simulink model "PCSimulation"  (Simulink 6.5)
settings: Solver=FixedStepDiscrete  SolverMode=SingleTasking  StartTime=0.0  StopTime=inf  FixedStep=samplePeriod  RelTol=1e-3  AbsTol=1e-6
PreLoadFcn:
  | initialize
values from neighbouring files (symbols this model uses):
  actParams = [	bulkModulus   * pressCanon    [Copy of initialize.m]    (also in initialize.m = [bulkModulus	* pressCanon,)
  displFreq = inf    [initialize.m]
  flowCanon = 1.666667e+04    (= 16666.67)    [Copy of initialize.m]    (also in initialize.m)
  forceCanon = 1    [Copy of initialize.m]    (also in initialize.m)
  forceFreq = inf    [initialize.m]
  friction = 5			 				* 0.155000	 				* 0.00444822 				* area1    (= 2.71252900422)    [initialize.m]
  fsamp = 1 / samplePeriod    (= 1024)    [Copy of initialize.m]    (also in initialize.m; rampth.m = 1 / deltaT; randth.m = 1 / deltaT; rspect.m = 1.0 / tsamp)
  gasConstant = 1.8    [Copy of initialize.m]    (also in initialize.m)
  lengthCanon = 1    [Copy of initialize.m]    (also in initialize.m)
  massCanon = 1e-06    [Copy of initialize.m]    (also in initialize.m)
  maxDispl = ( (stroke2 + endLength2) * lengthCanon)'    [Copy of initialize.m]    (also in initialize.m = 576.2)
  maxOilVolume = volume * (1 - (precharge/supplyPress)^(1/gasConstant))    (= 211.391477114)    [Copy of initialize.m]    (also in initialize.m)
  maxVeloc = ( (maxFlow' * flowCanon ./ (area1 * areaCanon)) / velocCanon)'    [Copy of initialize.m]    (also in initialize.m = (maxFlow * flowCanon / (area1 * areaCanon)) / velocCanon; rampth.m = 2 * maxDispl / (nVeloc * deltaT))
  minDispl = (-(stroke1 + endLength1) * lengthCanon)'    [Copy of initialize.m]    (also in initialize.m = -576.2)
  minVeloc = (-(maxFlow' * flowCanon ./ (area2 * areaCanon)) / velocCanon)'    [Copy of initialize.m]    (also in initialize.m = -(maxFlow * flowCanon / (area2 * areaCanon)) / velocCanon)
  nAct = 5    [Copy of initialize.m]    (also in initialize.m = 1)
  nAdcU = 6    [Copy of initialize.m]    (also in initialize.m = 5)
  nDinp = 4    [Copy of initialize.m]    (also in initialize.m)
  nDout = 4    [Copy of initialize.m]    (also in initialize.m)
  nDucU = 2    [Copy of initialize.m]    (also in initialize.m)
  nEncU = 3    [Copy of initialize.m]    (also in initialize.m)
  nUDPInp = 1+6*nAct+nAdcU+nDucU+nEncU+nDout    (= 46)    [Copy of initialize.m]    (also in initialize.m = 10)
  nUDPOut = 1+7*nAct+nAdcU+nDucU+nEncU+nDinp    (= 51)    [Copy of initialize.m]    (also in initialize.m = 12)
  precharge = 3000		 				* 6.894757e-03    (= 20.684271)    [Copy of initialize.m]    (also in initialize.m)
  pumpFlow = 1e20    (= 1e+20)    [Copy of initialize.m]    (also in initialize.m)
  returnPress = 3			 				* 0.1    (= 0.3)    [Copy of initialize.m]    (also in initialize.m)
  samplePeriod = controlPeriod/upsampleFactor    (= 0.0009765625)    [Copy of initialize.m]    (also in initialize.m; viewer.m = eval(getHeaderValue(header, 'DELTA_T')))
  springCanon = 1    [Copy of initialize.m]    (also in initialize.m)
  supplyPress = 280		 				* 0.1    (= 28)    [Copy of initialize.m]    (also in initialize.m)
  upsampleFactor = 1    [Copy of initialize.m]    (also in initialize.m)
  velocCanon = 1    [Copy of initialize.m]    (also in initialize.m)
  volume = 15.15		 				+ (  45		 				    * 2		 				   + 30		 				    * 6 )	 				* 5    (= 1365.15)    [Copy of initialize.m]    (also in initialize.m; quake.m = volume / 231.0)
  volumeCanon = 1e+06    (= 1000000)    [Copy of initialize.m]    (also in initialize.m)
  yieldDispl = 1.0    (= 1)    [initialize.m]
undefined symbols (not defined in the file or in its folder): DiscIntNeverNeededParam, dpforceFreq, mass, spring, staticForce
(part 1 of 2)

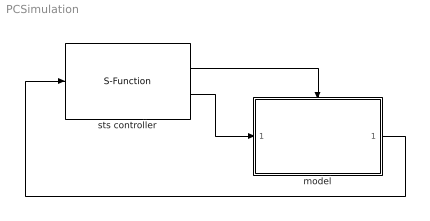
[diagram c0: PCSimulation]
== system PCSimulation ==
  model : Subsystem  TreatAsAtomicUnit=on
  sts controller : S-Function  FunctionName=ConnectUdpSimulink  Parameters=5002,nUDPInp,nUDPOut,upsampleFactor
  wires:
  model/1(out) -> sts controller/1
  sts controller/1 -> model/Trigger
  sts controller/2 -> model/1(inp)

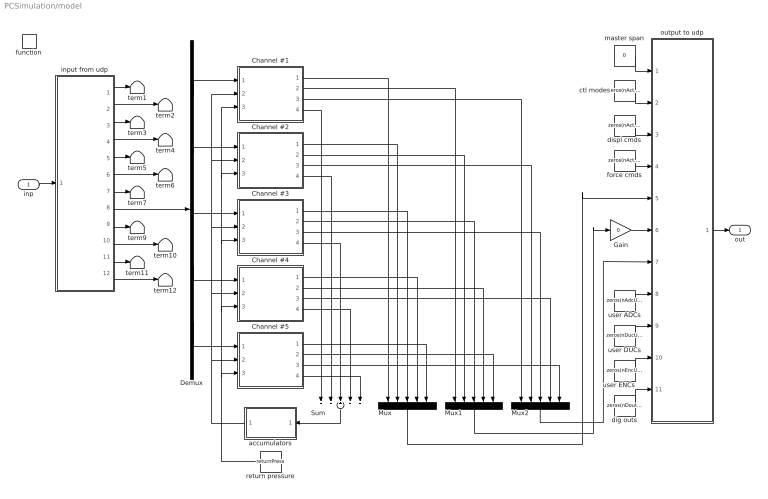
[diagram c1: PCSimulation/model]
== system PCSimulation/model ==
  inp : Inport
  function : TriggerPort  TriggerType=function-call
  Channel #1 : Subsystem  mask{id=1}
      mask prompts: id "Channel ID"
  Channel #2 : Subsystem  mask{id=2}
      mask prompts: id "Channel ID"
  Channel #3 : Subsystem  mask{id=3}
      mask prompts: id "Channel ID"
  Channel #4 : Subsystem  mask{id=4}
      mask prompts: id "Channel ID"
  Channel #5 : Subsystem  mask{id=5}
      mask prompts: id "Channel ID"
  Demux : Demux  Outputs=nAct
  Gain : Gain  Gain=0
  Mux : Mux  Orientation=down  Inputs=nAct
  Mux1 : Mux  Orientation=down  Inputs=nAct
  Mux2 : Mux  Orientation=down  Inputs=nAct
  Sum : Sum  Orientation=down  Inputs=+++++
  accumulators : Subsystem  Orientation=left
  ctl modes : Constant  Value=zeros(nAct, 1)  OutDataType=sfix(16)  ConRadixGroup=Use specified scaling  OutScaling=2^0  SampleTime=inf  FramePeriod=inf
  dig outs : Constant  Value=zeros(nDout, 1)  OutDataTypeMode=uint32  OutDataType=sfix(16)  ConRadixGroup=Use specified scaling  OutScaling=2^0  SampleTime=inf  FramePeriod=inf
  displ cmds : Constant  Value=zeros(nAct, 1)  OutDataType=sfix(16)  ConRadixGroup=Use specified scaling  OutScaling=2^0  SampleTime=inf  FramePeriod=inf
  force cmds : Constant  Value=zeros(nAct, 1)  OutDataType=sfix(16)  ConRadixGroup=Use specified scaling  OutScaling=2^0  SampleTime=inf  FramePeriod=inf
  input from udp : Subsystem
  master span : Constant  Value=0  OutDataType=sfix(16)  ConRadixGroup=Use specified scaling  OutScaling=2^0  SampleTime=inf  FramePeriod=inf
  output to udp : Subsystem
  return pressure : Constant  Orientation=left  Value=returnPress  OutDataType=sfix(16)  ConRadixGroup=Use specified scaling  OutScaling=2^0  SampleTime=inf  FramePeriod=inf
  term{1..7,9..12} (11 alike) : Terminator
  user ADCs : Constant  Value=zeros(nAdcU, 1)  OutDataType=sfix(16)  ConRadixGroup=Use specified scaling  OutScaling=2^0  SampleTime=inf  FramePeriod=inf
  user DUCs : Constant  Value=zeros(nDucU, 1)  OutDataType=sfix(16)  ConRadixGroup=Use specified scaling  OutScaling=2^0  SampleTime=inf  FramePeriod=inf
  user ENCs : Constant  Value=zeros(nEncU, 1)  OutDataType=sfix(16)  ConRadixGroup=Use specified scaling  OutScaling=2^0  SampleTime=inf  FramePeriod=inf
  out : Outport
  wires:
  input from udp/3(displ cmds) -> term3/1
  input from udp/1(master span) -> term1/1
  input from udp/6(force fbks) -> term6/1
  input from udp/10(user ducs) -> term10/1
  input from udp/12(dig inps) -> term12/1
  input from udp/2(ctl modes) -> term2/1
  input from udp/4(force cmds) -> term4/1
  input from udp/5(displ fbks) -> term5/1
  input from udp/7(dpforce fbks) -> term7/1
  input from udp/9(user adcs) -> term9/1
  input from udp/11(user encs) -> term11/1
  inp/1 -> input from udp/1(inp)
  master span/1 -> output to udp/1(master span)
  ctl modes/1 -> output to udp/2(ctl modes)
  displ cmds/1 -> output to udp/3(displ cmds)
  force cmds/1 -> output to udp/4(force cmds)
  user ADCs/1 -> output to udp/8(user adcs)
  user DUCs/1 -> output to udp/9(user ducs)
  user ENCs/1 -> output to udp/10(user encs)
  dig outs/1 -> output to udp/11(dig outs)
  output to udp/1(out) -> out/1
  Channel #1/4(flow) -> Sum/1
  Channel #2/4(flow) -> Sum/2
  Channel #3/4(flow) -> Sum/3
  Sum/1 -> accumulators/1(flow)
  Channel #4/4(flow) -> Sum/4
  Channel #5/4(flow) -> Sum/5
  Channel #1/1(displ) -> Mux/1
  Channel #2/1(displ) -> Mux/2
  Channel #3/1(displ) -> Mux/3
  Channel #4/1(displ) -> Mux/4
  Channel #5/1(displ) -> Mux/5
  Channel #1/2(force) -> Mux1/1
  Channel #2/2(force) -> Mux1/2
  Channel #3/2(force) -> Mux1/3
  Channel #4/2(force) -> Mux1/4
  Channel #5/2(force) -> Mux1/5
  Channel #1/3(dpforce) -> Mux2/1
  Channel #2/3(dpforce) -> Mux2/2
  Channel #3/3(dpforce) -> Mux2/3
  Channel #4/3(dpforce) -> Mux2/4
  Channel #5/3(dpforce) -> Mux2/5
  Mux/1 -> output to udp/5(displ fbks)
  Mux1/1 -> Gain/1
  Mux2/1 -> output to udp/7(dpforce fbks)
  input from udp/8(valve cmds) -> Demux/1
  Demux/1 -> Channel #1/1(valve cmd)
  Demux/2 -> Channel #2/1(valve cmd)
  Demux/3 -> Channel #3/1(valve cmd)
  Demux/4 -> Channel #4/1(valve cmd)
  Demux/5 -> Channel #5/1(valve cmd)
  accumulators/1(press) -> Channel #1/2(spl press), Channel #2/2(spl press), Channel #3/2(spl press), Channel #4/2(spl press), Channel #5/2(spl press)
  return pressure/1 -> Channel #1/3(rtn press), Channel #2/3(rtn press), Channel #3/3(rtn press), Channel #4/3(rtn press), Channel #5/3(rtn press)
  Gain/1 -> output to udp/6(force fbks)

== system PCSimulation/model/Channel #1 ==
  valve cmd : Inport
  spl press : Inport  Port=2
  rtn press : Inport  Port=3
  displ cond filter : Subsystem  mask{freq3dB=displFreq(id), fsamp=fsamp}
      mask prompts: freq3dB "3 dB cutoff frequency (inf, 500, 300, 100, 50 Hz)"; fsamp "Sampling frequency (Hz)"
      mask init:
      | if isempty(freq3dB)
      | 	freq3dB = fsamp;
      | elseif freq3dB == 500
      | 	freq3dB = 485;
      | elseif freq3dB == 300
      | 	freq3dB = 204.9;
      | elseif freq3dB == 100
      | 	freq3dB = 56.5;
      | elseif freq3dB == 50
      | 	freq3dB = 27.8;
      | else
      | 	freq3dB = fsamp;
      | end
      | if freq3dB > fsamp/2
      | 	a = [1];
      | 	b = [1];
      | else
      | 	[b, a] = ellip(4, 0.001, 60.0, 2*freq3dB/fsamp);
      | end
  dpforce cond filter : Subsystem  mask{freq3dB=dpforceFreq(id), fsamp=fsamp}
      mask prompts: freq3dB "3 dB cutoff frequency (inf, 500, 300, 100, 50 Hz)"; fsamp "Sampling frequency (Hz)"
      mask init:
      | if isempty(freq3dB)
      | 	freq3dB = fsamp;
      | elseif freq3dB == 500
      | 	freq3dB = 485;
      | elseif freq3dB == 300
      | 	freq3dB = 204.9;
      | elseif freq3dB == 100
      | 	freq3dB = 56.5;
      | elseif freq3dB == 50
      | 	freq3dB = 27.8;
      | else
      | 	freq3dB = fsamp;
      | end
      | if freq3dB > fsamp/2
      | 	a = [1];
      | 	b = [1];
      | else
      | 	[b, a] = ellip(4, 0.001, 60.0, 2*freq3dB/fsamp);
      | end
  force cond filter : Subsystem  mask{freq3dB=forceFreq((id)), fsamp=fsamp}
      mask prompts: freq3dB "3 dB cutoff frequency (inf, 500, 300, 100, 50 Hz)"; fsamp "Sampling frequency (Hz)"
      mask init:
      | if isempty(freq3dB)
      | 	freq3dB = fsamp;
      | elseif freq3dB == 500
      | 	freq3dB = 485;
      | elseif freq3dB == 300
      | 	freq3dB = 204.9;
      | elseif freq3dB == 100
      | 	freq3dB = 56.5;
      | elseif freq3dB == 50
      | 	freq3dB = 27.8;
      | else
      | 	freq3dB = fsamp;
      | end
      | if freq3dB > fsamp/2
      | 	a = [1];
      | 	b = [1];
      | else
      | 	[b, a] = ellip(4, 0.001, 60.0, 2*freq3dB/fsamp);
      | end
  payload : Subsystem
  servovalve & actuator : Subsystem  mask(Actuator){params=actParams(:,id)}
      mask prompts: params "Parameter vector"
  displ : Outport
  force : Outport  Port=2
  dpforce : Outport  Port=3
  flow : Outport  Port=4
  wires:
  payload/2(veloc) -> servovalve & actuator/3(veloc)
  payload/1(displ) -> displ cond filter/1(inp), servovalve & actuator/2(displ)
  valve cmd/1 -> servovalve & actuator/1(cmd)
  rtn press/1 -> servovalve & actuator/5(rtn press)
  spl press/1 -> servovalve & actuator/4(spl press)
  servovalve & actuator/2(flow) -> flow/1
  servovalve & actuator/1(force) -> force cond filter/1(inp), dpforce cond filter/1(inp), payload/1(force)
  displ cond filter/1(out) -> displ/1
  force cond filter/1(out) -> force/1
  dpforce cond filter/1(out) -> dpforce/1

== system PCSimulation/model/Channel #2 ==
  valve cmd : Inport
  spl press : Inport  Port=2
  rtn press : Inport  Port=3
  displ cond filter : Subsystem  mask{freq3dB=displFreq(id), fsamp=fsamp}
      mask prompts: freq3dB "3 dB cutoff frequency (inf, 500, 300, 100, 50 Hz)"; fsamp "Sampling frequency (Hz)"
      mask init:
      | if isempty(freq3dB)
      | 	freq3dB = fsamp;
      | elseif freq3dB == 500
      | 	freq3dB = 485;
      | elseif freq3dB == 300
      | 	freq3dB = 204.9;
      | elseif freq3dB == 100
      | 	freq3dB = 56.5;
      | elseif freq3dB == 50
      | 	freq3dB = 27.8;
      | else
      | 	freq3dB = fsamp;
      | end
      | if freq3dB > fsamp/2
      | 	a = [1];
      | 	b = [1];
      | else
      | 	[b, a] = ellip(4, 0.001, 60.0, 2*freq3dB/fsamp);
      | end
  dpforce cond filter : Subsystem  mask{freq3dB=dpforceFreq(id), fsamp=fsamp}
      mask prompts: freq3dB "3 dB cutoff frequency (inf, 500, 300, 100, 50 Hz)"; fsamp "Sampling frequency (Hz)"
      mask init:
      | if isempty(freq3dB)
      | 	freq3dB = fsamp;
      | elseif freq3dB == 500
      | 	freq3dB = 485;
      | elseif freq3dB == 300
      | 	freq3dB = 204.9;
      | elseif freq3dB == 100
      | 	freq3dB = 56.5;
      | elseif freq3dB == 50
      | 	freq3dB = 27.8;
      | else
      | 	freq3dB = fsamp;
      | end
      | if freq3dB > fsamp/2
      | 	a = [1];
      | 	b = [1];
      | else
      | 	[b, a] = ellip(4, 0.001, 60.0, 2*freq3dB/fsamp);
      | end
  force cond filter : Subsystem  mask{freq3dB=forceFreq((id)), fsamp=fsamp}
      mask prompts: freq3dB "3 dB cutoff frequency (inf, 500, 300, 100, 50 Hz)"; fsamp "Sampling frequency (Hz)"
      mask init:
      | if isempty(freq3dB)
      | 	freq3dB = fsamp;
      | elseif freq3dB == 500
      | 	freq3dB = 485;
      | elseif freq3dB == 300
      | 	freq3dB = 204.9;
      | elseif freq3dB == 100
      | 	freq3dB = 56.5;
      | elseif freq3dB == 50
      | 	freq3dB = 27.8;
      | else
      | 	freq3dB = fsamp;
      | end
      | if freq3dB > fsamp/2
      | 	a = [1];
      | 	b = [1];
      | else
      | 	[b, a] = ellip(4, 0.001, 60.0, 2*freq3dB/fsamp);
      | end
  payload : Subsystem
  servovalve & actuator : Subsystem  mask(Actuator){params=actParams(:,id)}
      mask prompts: params "Parameter vector"
  displ : Outport
  force : Outport  Port=2
  dpforce : Outport  Port=3
  flow : Outport  Port=4
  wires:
  dpforce cond filter/1(out) -> dpforce/1
  force cond filter/1(out) -> force/1
  displ cond filter/1(out) -> displ/1
  servovalve & actuator/1(force) -> payload/1(force), dpforce cond filter/1(inp), force cond filter/1(inp)
  servovalve & actuator/2(flow) -> flow/1
  spl press/1 -> servovalve & actuator/4(spl press)
  rtn press/1 -> servovalve & actuator/5(rtn press)
  valve cmd/1 -> servovalve & actuator/1(cmd)
  payload/1(displ) -> servovalve & actuator/2(displ), displ cond filter/1(inp)
  payload/2(veloc) -> servovalve & actuator/3(veloc)

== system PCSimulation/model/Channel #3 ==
  valve cmd : Inport
  spl press : Inport  Port=2
  rtn press : Inport  Port=3
  displ cond filter : Subsystem  mask{freq3dB=displFreq(id), fsamp=fsamp}
      mask prompts: freq3dB "3 dB cutoff frequency (inf, 500, 300, 100, 50 Hz)"; fsamp "Sampling frequency (Hz)"
      mask init:
      | if isempty(freq3dB)
      | 	freq3dB = fsamp;
      | elseif freq3dB == 500
      | 	freq3dB = 485;
      | elseif freq3dB == 300
      | 	freq3dB = 204.9;
      | elseif freq3dB == 100
      | 	freq3dB = 56.5;
      | elseif freq3dB == 50
      | 	freq3dB = 27.8;
      | else
      | 	freq3dB = fsamp;
      | end
      | if freq3dB > fsamp/2
      | 	a = [1];
      | 	b = [1];
      | else
      | 	[b, a] = ellip(4, 0.001, 60.0, 2*freq3dB/fsamp);
      | end
  dpforce cond filter : Subsystem  mask{freq3dB=dpforceFreq(id), fsamp=fsamp}
      mask prompts: freq3dB "3 dB cutoff frequency (inf, 500, 300, 100, 50 Hz)"; fsamp "Sampling frequency (Hz)"
      mask init:
      | if isempty(freq3dB)
      | 	freq3dB = fsamp;
      | elseif freq3dB == 500
      | 	freq3dB = 485;
      | elseif freq3dB == 300
      | 	freq3dB = 204.9;
      | elseif freq3dB == 100
      | 	freq3dB = 56.5;
      | elseif freq3dB == 50
      | 	freq3dB = 27.8;
      | else
      | 	freq3dB = fsamp;
      | end
      | if freq3dB > fsamp/2
      | 	a = [1];
      | 	b = [1];
      | else
      | 	[b, a] = ellip(4, 0.001, 60.0, 2*freq3dB/fsamp);
      | end
  force cond filter : Subsystem  mask{freq3dB=forceFreq((id)), fsamp=fsamp}
      mask prompts: freq3dB "3 dB cutoff frequency (inf, 500, 300, 100, 50 Hz)"; fsamp "Sampling frequency (Hz)"
      mask init:
      | if isempty(freq3dB)
      | 	freq3dB = fsamp;
      | elseif freq3dB == 500
      | 	freq3dB = 485;
      | elseif freq3dB == 300
      | 	freq3dB = 204.9;
      | elseif freq3dB == 100
      | 	freq3dB = 56.5;
      | elseif freq3dB == 50
      | 	freq3dB = 27.8;
      | else
      | 	freq3dB = fsamp;
      | end
      | if freq3dB > fsamp/2
      | 	a = [1];
      | 	b = [1];
      | else
      | 	[b, a] = ellip(4, 0.001, 60.0, 2*freq3dB/fsamp);
      | end
  payload : Subsystem
  servovalve & actuator : Subsystem  mask(Actuator){params=actParams(:,id)}
      mask prompts: params "Parameter vector"
  displ : Outport
  force : Outport  Port=2
  dpforce : Outport  Port=3
  flow : Outport  Port=4
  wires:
  payload/2(veloc) -> servovalve & actuator/3(veloc)
  payload/1(displ) -> displ cond filter/1(inp), servovalve & actuator/2(displ)
  valve cmd/1 -> servovalve & actuator/1(cmd)
  rtn press/1 -> servovalve & actuator/5(rtn press)
  spl press/1 -> servovalve & actuator/4(spl press)
  servovalve & actuator/2(flow) -> flow/1
  servovalve & actuator/1(force) -> force cond filter/1(inp), dpforce cond filter/1(inp), payload/1(force)
  displ cond filter/1(out) -> displ/1
  force cond filter/1(out) -> force/1
  dpforce cond filter/1(out) -> dpforce/1

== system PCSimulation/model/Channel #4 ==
  valve cmd : Inport
  spl press : Inport  Port=2
  rtn press : Inport  Port=3
  displ cond filter : Subsystem  mask{freq3dB=displFreq(id), fsamp=fsamp}
      mask prompts: freq3dB "3 dB cutoff frequency (inf, 500, 300, 100, 50 Hz)"; fsamp "Sampling frequency (Hz)"
      mask init:
      | if isempty(freq3dB)
      | 	freq3dB = fsamp;
      | elseif freq3dB == 500
      | 	freq3dB = 485;
      | elseif freq3dB == 300
      | 	freq3dB = 204.9;
      | elseif freq3dB == 100
      | 	freq3dB = 56.5;
      | elseif freq3dB == 50
      | 	freq3dB = 27.8;
      | else
      | 	freq3dB = fsamp;
      | end
      | if freq3dB > fsamp/2
      | 	a = [1];
      | 	b = [1];
      | else
      | 	[b, a] = ellip(4, 0.001, 60.0, 2*freq3dB/fsamp);
      | end
  dpforce cond filter : Subsystem  mask{freq3dB=dpforceFreq(id), fsamp=fsamp}
      mask prompts: freq3dB "3 dB cutoff frequency (inf, 500, 300, 100, 50 Hz)"; fsamp "Sampling frequency (Hz)"
      mask init:
      | if isempty(freq3dB)
      | 	freq3dB = fsamp;
      | elseif freq3dB == 500
      | 	freq3dB = 485;
      | elseif freq3dB == 300
      | 	freq3dB = 204.9;
      | elseif freq3dB == 100
      | 	freq3dB = 56.5;
      | elseif freq3dB == 50
      | 	freq3dB = 27.8;
      | else
      | 	freq3dB = fsamp;
      | end
      | if freq3dB > fsamp/2
      | 	a = [1];
      | 	b = [1];
      | else
      | 	[b, a] = ellip(4, 0.001, 60.0, 2*freq3dB/fsamp);
      | end
  force cond filter : Subsystem  mask{freq3dB=forceFreq((id)), fsamp=fsamp}
      mask prompts: freq3dB "3 dB cutoff frequency (inf, 500, 300, 100, 50 Hz)"; fsamp "Sampling frequency (Hz)"
      mask init:
      | if isempty(freq3dB)
      | 	freq3dB = fsamp;
      | elseif freq3dB == 500
      | 	freq3dB = 485;
      | elseif freq3dB == 300
      | 	freq3dB = 204.9;
      | elseif freq3dB == 100
      | 	freq3dB = 56.5;
      | elseif freq3dB == 50
      | 	freq3dB = 27.8;
      | else
      | 	freq3dB = fsamp;
      | end
      | if freq3dB > fsamp/2
      | 	a = [1];
      | 	b = [1];
      | else
      | 	[b, a] = ellip(4, 0.001, 60.0, 2*freq3dB/fsamp);
      | end
  payload : Subsystem
  servovalve & actuator : Subsystem  mask(Actuator){params=actParams(:,id)}
      mask prompts: params "Parameter vector"
  displ : Outport
  force : Outport  Port=2
  dpforce : Outport  Port=3
  flow : Outport  Port=4
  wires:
  dpforce cond filter/1(out) -> dpforce/1
  force cond filter/1(out) -> force/1
  displ cond filter/1(out) -> displ/1
  servovalve & actuator/1(force) -> payload/1(force), dpforce cond filter/1(inp), force cond filter/1(inp)
  servovalve & actuator/2(flow) -> flow/1
  spl press/1 -> servovalve & actuator/4(spl press)
  rtn press/1 -> servovalve & actuator/5(rtn press)
  valve cmd/1 -> servovalve & actuator/1(cmd)
  payload/1(displ) -> servovalve & actuator/2(displ), displ cond filter/1(inp)
  payload/2(veloc) -> servovalve & actuator/3(veloc)

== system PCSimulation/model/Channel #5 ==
  valve cmd : Inport
  spl press : Inport  Port=2
  rtn press : Inport  Port=3
  displ cond filter : Subsystem  mask{freq3dB=displFreq(id), fsamp=fsamp}
      mask prompts: freq3dB "3 dB cutoff frequency (inf, 500, 300, 100, 50 Hz)"; fsamp "Sampling frequency (Hz)"
      mask init:
      | if isempty(freq3dB)
      | 	freq3dB = fsamp;
      | elseif freq3dB == 500
      | 	freq3dB = 485;
      | elseif freq3dB == 300
      | 	freq3dB = 204.9;
      | elseif freq3dB == 100
      | 	freq3dB = 56.5;
      | elseif freq3dB == 50
      | 	freq3dB = 27.8;
      | else
      | 	freq3dB = fsamp;
      | end
      | if freq3dB > fsamp/2
      | 	a = [1];
      | 	b = [1];
      | else
      | 	[b, a] = ellip(4, 0.001, 60.0, 2*freq3dB/fsamp);
      | end
  dpforce cond filter : Subsystem  mask{freq3dB=dpforceFreq(id), fsamp=fsamp}
      mask prompts: freq3dB "3 dB cutoff frequency (inf, 500, 300, 100, 50 Hz)"; fsamp "Sampling frequency (Hz)"
      mask init:
      | if isempty(freq3dB)
      | 	freq3dB = fsamp;
      | elseif freq3dB == 500
      | 	freq3dB = 485;
      | elseif freq3dB == 300
      | 	freq3dB = 204.9;
      | elseif freq3dB == 100
      | 	freq3dB = 56.5;
      | elseif freq3dB == 50
      | 	freq3dB = 27.8;
      | else
      | 	freq3dB = fsamp;
      | end
      | if freq3dB > fsamp/2
      | 	a = [1];
      | 	b = [1];
      | else
      | 	[b, a] = ellip(4, 0.001, 60.0, 2*freq3dB/fsamp);
      | end
  force cond filter : Subsystem  mask{freq3dB=forceFreq((id)), fsamp=fsamp}
      mask prompts: freq3dB "3 dB cutoff frequency (inf, 500, 300, 100, 50 Hz)"; fsamp "Sampling frequency (Hz)"
      mask init:
      | if isempty(freq3dB)
      | 	freq3dB = fsamp;
      | elseif freq3dB == 500
      | 	freq3dB = 485;
      | elseif freq3dB == 300
      | 	freq3dB = 204.9;
      | elseif freq3dB == 100
      | 	freq3dB = 56.5;
      | elseif freq3dB == 50
      | 	freq3dB = 27.8;
      | else
      | 	freq3dB = fsamp;
      | end
      | if freq3dB > fsamp/2
      | 	a = [1];
      | 	b = [1];
      | else
      | 	[b, a] = ellip(4, 0.001, 60.0, 2*freq3dB/fsamp);
      | end
  payload : Subsystem
  servovalve & actuator : Subsystem  mask(Actuator){params=actParams(:,id)}
      mask prompts: params "Parameter vector"
  displ : Outport
  force : Outport  Port=2
  dpforce : Outport  Port=3
  flow : Outport  Port=4
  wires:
  payload/2(veloc) -> servovalve & actuator/3(veloc)
  payload/1(displ) -> displ cond filter/1(inp), servovalve & actuator/2(displ)
  valve cmd/1 -> servovalve & actuator/1(cmd)
  rtn press/1 -> servovalve & actuator/5(rtn press)
  spl press/1 -> servovalve & actuator/4(spl press)
  servovalve & actuator/2(flow) -> flow/1
  servovalve & actuator/1(force) -> force cond filter/1(inp), dpforce cond filter/1(inp), payload/1(force)
  displ cond filter/1(out) -> displ/1
  force cond filter/1(out) -> force/1
  dpforce cond filter/1(out) -> dpforce/1

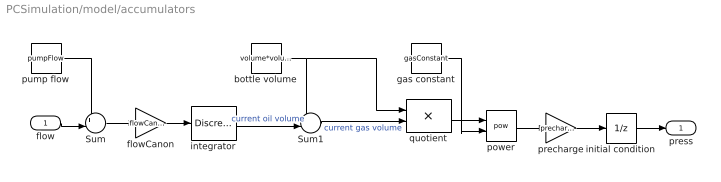
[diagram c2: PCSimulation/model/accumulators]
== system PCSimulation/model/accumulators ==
  flow : Inport
  Sum : Sum  Inputs=+-|
  Sum1 : Sum  Inputs=+-|
  bottle volume : Constant  Value=volume*volumeCanon  OutDataType=sfix(16)  ConRadixGroup=Use specified scaling  OutScaling=2^0  SampleTime=inf  FramePeriod=inf
  flowCanon : Gain  Gain=flowCanon
  gas constant : Constant  Value=gasConstant  OutDataType=sfix(16)  ConRadixGroup=Use specified scaling  OutScaling=2^0  SampleTime=inf  FramePeriod=inf
  initial condition : UnitDelay  X0=supplyPress  SampleTime=-1
  integrator : DiscreteIntegrator  InitialCondition=maxOilVolume*volumeCanon  SampleTime=-1  LimitOutput=on  UpperSaturationLimit=maxOilVolume*volumeCanon  LowerSaturationLimit=0  ICPrevOutput=DiscIntNeverNeededParam  ICPrevScaledInput=DiscIntNeverNeededParam
  power : Math  Operator=pow
  precharge : Gain  Gain=precharge
  pump flow : Constant  Value=pumpFlow  OutDataType=sfix(16)  ConRadixGroup=Use specified scaling  OutScaling=2^0  SampleTime=inf  FramePeriod=inf
  quotient : Product  Inputs=*/
  press : Outport
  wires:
  initial condition/1 -> press/1
  flowCanon/1 -> integrator/1
  flow/1 -> Sum/2
  integrator/1 -> Sum1/2  "current oil volume"
  quotient/1 -> power/1
  Sum1/1 -> quotient/2  "current gas volume"
  precharge/1 -> initial condition/1
  power/1 -> precharge/1
  gas constant/1 -> power/2
  bottle volume/1 -> quotient/1, Sum1/1
  Sum/1 -> flowCanon/1
  pump flow/1 -> Sum/1

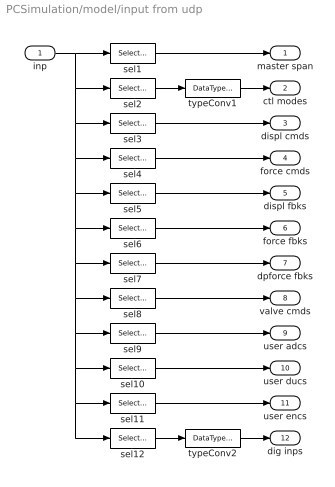
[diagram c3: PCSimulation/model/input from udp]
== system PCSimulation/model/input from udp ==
  inp : Inport
  sel1 : Selector  InputType=Vector  ElementSrc=Internal  Elements=[0]+1  RowSrc=Internal  Rows=1  ColumnSrc=Internal  Columns=1  InputPortWidth=nUDPOut  IndexIsStartValue=off
  sel10 : Selector  InputType=Vector  ElementSrc=Internal  Elements=[1:nDucU]+1+7*nAct+nAdcU  RowSrc=Internal  Rows=1  ColumnSrc=Internal  Columns=1  InputPortWidth=nUDPOut  IndexIsStartValue=off
  sel11 : Selector  InputType=Vector  ElementSrc=Internal  Elements=[1:nEncU]+1+7*nAct+nAdcU+nDucU  RowSrc=Internal  Rows=1  ColumnSrc=Internal  Columns=1  InputPortWidth=nUDPOut  IndexIsStartValue=off
  sel12 : Selector  InputType=Vector  ElementSrc=Internal  Elements=[1:nDinp]+1+7*nAct+nAdcU+nDucU+nEncU  RowSrc=Internal  Rows=1  ColumnSrc=Internal  Columns=1  InputPortWidth=nUDPOut  IndexIsStartValue=off
  sel2 : Selector  InputType=Vector  ElementSrc=Internal  Elements=[1:nAct]+1+0*nAct  RowSrc=Internal  Rows=1  ColumnSrc=Internal  Columns=1  InputPortWidth=nUDPOut  IndexIsStartValue=off
  sel3 : Selector  InputType=Vector  ElementSrc=Internal  Elements=[1:nAct]+1+1*nAct  RowSrc=Internal  Rows=1  ColumnSrc=Internal  Columns=1  InputPortWidth=nUDPOut  IndexIsStartValue=off
  sel4 : Selector  InputType=Vector  ElementSrc=Internal  Elements=[1:nAct]+1+2*nAct  RowSrc=Internal  Rows=1  ColumnSrc=Internal  Columns=1  InputPortWidth=nUDPOut  IndexIsStartValue=off
  sel5 : Selector  InputType=Vector  ElementSrc=Internal  Elements=[1:nAct]+1+3*nAct  RowSrc=Internal  Rows=1  ColumnSrc=Internal  Columns=1  InputPortWidth=nUDPOut  IndexIsStartValue=off
  sel6 : Selector  InputType=Vector  ElementSrc=Internal  Elements=[1:nAct]+1+4*nAct  RowSrc=Internal  Rows=1  ColumnSrc=Internal  Columns=1  InputPortWidth=nUDPOut  IndexIsStartValue=off
  sel7 : Selector  InputType=Vector  ElementSrc=Internal  Elements=[1:nAct]+1+5*nAct  RowSrc=Internal  Rows=1  ColumnSrc=Internal  Columns=1  InputPortWidth=nUDPOut  IndexIsStartValue=off
  sel8 : Selector  InputType=Vector  ElementSrc=Internal  Elements=[1:nAct]+1+6*nAct  RowSrc=Internal  Rows=1  ColumnSrc=Internal  Columns=1  InputPortWidth=nUDPOut  IndexIsStartValue=off
  sel9 : Selector  InputType=Vector  ElementSrc=Internal  Elements=[1:nAdcU]+1+7*nAct  RowSrc=Internal  Rows=1  ColumnSrc=Internal  Columns=1  InputPortWidth=nUDPOut  IndexIsStartValue=off
  typeConv1 : DataTypeConversion  OutDataTypeMode=uint32
  typeConv2 : DataTypeConversion  OutDataTypeMode=uint32
  master span : Outport
  ctl modes : Outport  Port=2
  displ cmds : Outport  Port=3
  force cmds : Outport  Port=4
  displ fbks : Outport  Port=5
  force fbks : Outport  Port=6
  dpforce fbks : Outport  Port=7
  valve cmds : Outport  Port=8
  user adcs : Outport  Port=9
  user ducs : Outport  Port=10
  user encs : Outport  Port=11
  dig inps : Outport  Port=12
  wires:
  sel1/1 -> master span/1
  sel2/1 -> typeConv1/1
  sel3/1 -> displ cmds/1
  sel4/1 -> force cmds/1
  sel5/1 -> displ fbks/1
  sel6/1 -> force fbks/1
  sel7/1 -> dpforce fbks/1
  sel8/1 -> valve cmds/1
  sel9/1 -> user adcs/1
  sel10/1 -> user ducs/1
  sel11/1 -> user encs/1
  sel12/1 -> typeConv2/1
  inp/1 -> sel1/1, sel2/1, sel3/1, sel11/1, sel12/1, sel10/1, sel9/1, sel8/1, sel7/1, sel6/1, sel5/1, sel4/1
  typeConv1/1 -> ctl modes/1
  typeConv2/1 -> dig inps/1

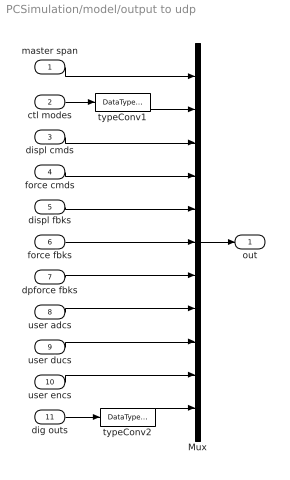
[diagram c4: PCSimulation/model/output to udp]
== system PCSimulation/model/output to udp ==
  master span : Inport
  ctl modes : Inport  Port=2
  displ cmds : Inport  Port=3
  force cmds : Inport  Port=4
  displ fbks : Inport  Port=5
  force fbks : Inport  Port=6
  dpforce fbks : Inport  Port=7
  user adcs : Inport  Port=8
  user ducs : Inport  Port=9
  user encs : Inport  Port=10
  dig outs : Inport  Port=11
  Mux : Mux  Inputs=11
  typeConv1 : DataTypeConversion  OutDataTypeMode=double
  typeConv2 : DataTypeConversion  OutDataTypeMode=double
  out : Outport
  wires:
  typeConv2/1 -> Mux/11
  dig outs/1 -> typeConv2/1
  user encs/1 -> Mux/10
  user ducs/1 -> Mux/9
  user adcs/1 -> Mux/8
  dpforce fbks/1 -> Mux/7
  force fbks/1 -> Mux/6
  displ fbks/1 -> Mux/5
  force cmds/1 -> Mux/4
  master span/1 -> Mux/1
  displ cmds/1 -> Mux/3
  ctl modes/1 -> typeConv1/1
  Mux/1 -> out/1
  typeConv1/1 -> Mux/2

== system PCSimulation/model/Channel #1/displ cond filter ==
  inp : Inport
  filter : DiscreteFilter  Numerator=b  Denominator=a  SampleTime=-1
  out : Outport
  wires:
  inp/1 -> filter/1
  filter/1 -> out/1

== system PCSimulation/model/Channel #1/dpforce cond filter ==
  inp : Inport
  filter : DiscreteFilter  Numerator=b  Denominator=a  SampleTime=-1
  out : Outport
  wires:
  filter/1 -> out/1
  inp/1 -> filter/1

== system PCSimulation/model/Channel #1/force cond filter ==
  inp : Inport
  filter : DiscreteFilter  Numerator=b  Denominator=a  SampleTime=-1
  out : Outport
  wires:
  inp/1 -> filter/1
  filter/1 -> out/1

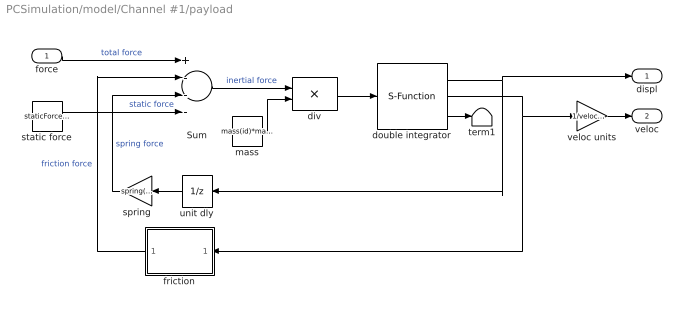
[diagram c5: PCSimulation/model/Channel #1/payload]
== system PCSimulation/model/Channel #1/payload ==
  force : Inport
  Sum : Sum  Inputs=+---
  div : Product  Inputs=*/
  double integrator : S-Function  FunctionName=doubleintegrator  Parameters=maxDispl, minDispl, initDispl, maxVeloc, minVeloc, initVeloc, samplePeriod  mask(Double integrator){maxDispl=maxDispl(id), minDispl=minDispl(id), initDispl=0, maxVeloc=maxVeloc(id)*velocCanon, minVeloc=minVeloc(id)*velocCanon, initVeloc=0, samplePeriod=samplePeriod}
      mask prompts: maxDispl "Maximum displacement"; minDispl "Minimum displacement"; initDispl "Initial displacement"; maxVeloc "Maximum velocity"; minVeloc "Minimum velocity"; initVeloc "Initial velocity"; samplePeriod "Sample period (sec)"
      mask help: Integrates acceleration twice to produce velocity and displacement. When clipping occurs, acceleration, velocity and displacement are adjusted accordingly.
  friction : Subsystem  Orientation=left  mask{friction=friction(id)*forceCanon, yieldDispl=yieldDispl(id)*lengthCanon, hysteresis=0}
      mask prompts: friction "Sliding friction"; yieldDispl "Equiv. yield displacement (in)"; hysteresis "Hysteresis constant"
  mass : Constant  Value=mass(id)*massCanon  OutDataType=sfix(16)  ConRadixGroup=Use specified scaling  OutScaling=2^0  SampleTime=inf  FramePeriod=inf
  spring : Gain  Orientation=left  Gain=spring(id)*springCanon
  static force : Constant  Value=staticForce(id)*forceCanon  OutDataType=sfix(16)  ConRadixGroup=Use specified scaling  OutScaling=2^0  SampleTime=inf  FramePeriod=inf
  term1 : Terminator
  unit dly : UnitDelay  Orientation=left  SampleTime=-1
  veloc units : Gain  Gain=1/velocCanon
  displ : Outport
  veloc : Outport  Port=2
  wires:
  friction/1(force) -> Sum/2  "friction force"
  unit dly/1 -> spring/1
  veloc units/1 -> veloc/1
  Sum/1 -> div/1  "inertial force"
  static force/1 -> Sum/4  "static force"
  force/1 -> Sum/1  "total force"
  mass/1 -> div/2
  spring/1 -> Sum/3  "spring force"
  double integrator/3 -> term1/1
  div/1 -> double integrator/1
  double integrator/1 -> displ/1, unit dly/1
  double integrator/2 -> veloc units/1, friction/1(veloc)

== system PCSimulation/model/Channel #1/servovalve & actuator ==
  note: Auxiliary diagnostic output vector: 1: valve opening 2: C1 pressure 3: C2 pressure 4: delta pressure 5: force 6: velocity 7: C1 flow 8: C2 flow 9: total flow 10: kinematic flow 11: compressibility flow 12: leakage flow 13: C1 oilspring displacement 14: C2 oilspring displacement 15: C1 oilspring velocity 16: C2 oilspring velocity
  note: Note: "1" and "2" denote actuator cylinders on either side of the actuator piston. With positive valve drive, oil is ported into cylinder 1, resulting in positive displacement.
  note: Parameter vector: 1: oil bulk modulus (force/displ^2) 2: servovalve delay (sec) 3: servovalve overlap 4: rated pressure (force/displ^2) 5: rated flow at rated pressure (displ^3/sec) 6: nominal flow at rated pressure (displ^3/sec) 7: actuator piston area 1 (displ^2) 8: actuator piston area 2 (displ^2) 9: actuator usable stroke 1 (displ) 10: actuator usable stroke 2 (displ) 11: actuator end cushion length 1 (displ) 12: actuator end cushion length 2 (displ) 13: additional port volume 1 (displ^3) 14: additional port volume 1 (displ^3) 15: actuator parasitic damping factor 16: cross-chamber leakage factor (flow/press) 17: ratio port openings according to area 18: sample period (sec) Conversion factors used for converting signals from external (user) to internal (canonical) units: 19: displacement 20: velocity 21: force 22: pressure 23: flow
  cmd : Inport
  displ : Inport  Port=2
  veloc : Inport  Port=3
  spl press : Inport  Port=4
  rtn press : Inport  Port=5
  abs : Abs  SaturateOnIntegerOverflow=on  SampleTime=-1
  actuator : S-Function  FunctionName=Actuator  Parameters=params
  total flow sel : Selector  InputType=Vector  ElementSrc=Internal  Elements=9  RowSrc=Internal  Rows=1  ColumnSrc=Internal  Columns=1  IndexIsStartValue=off
  force : Outport
  flow : Outport  Port=2
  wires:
  abs/1 -> flow/1
  total flow sel/1 -> abs/1
  actuator/2 -> total flow sel/1
  veloc/1 -> actuator/3
  displ/1 -> actuator/2
  actuator/1 -> force/1
  cmd/1 -> actuator/1
  rtn press/1 -> actuator/5
  spl press/1 -> actuator/4

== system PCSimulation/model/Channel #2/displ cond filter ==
  inp : Inport
  filter : DiscreteFilter  Numerator=b  Denominator=a  SampleTime=-1
  out : Outport
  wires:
  filter/1 -> out/1
  inp/1 -> filter/1

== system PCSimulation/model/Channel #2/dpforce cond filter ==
  inp : Inport
  filter : DiscreteFilter  Numerator=b  Denominator=a  SampleTime=-1
  out : Outport
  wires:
  inp/1 -> filter/1
  filter/1 -> out/1

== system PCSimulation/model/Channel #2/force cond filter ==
  inp : Inport
  filter : DiscreteFilter  Numerator=b  Denominator=a  SampleTime=-1
  out : Outport
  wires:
  filter/1 -> out/1
  inp/1 -> filter/1

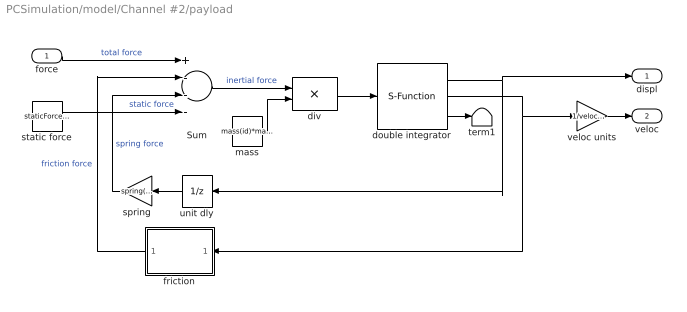
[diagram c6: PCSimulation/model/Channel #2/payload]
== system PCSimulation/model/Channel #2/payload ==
  force : Inport
  Sum : Sum  Inputs=+---
  div : Product  Inputs=*/
  double integrator : S-Function  FunctionName=doubleintegrator  Parameters=maxDispl, minDispl, initDispl, maxVeloc, minVeloc, initVeloc, samplePeriod  mask(Double integrator){maxDispl=maxDispl(id), minDispl=minDispl(id), initDispl=0, maxVeloc=maxVeloc(id)*velocCanon, minVeloc=minVeloc(id)*velocCanon, initVeloc=0, samplePeriod=samplePeriod}
      mask prompts: maxDispl "Maximum displacement"; minDispl "Minimum displacement"; initDispl "Initial displacement"; maxVeloc "Maximum velocity"; minVeloc "Minimum velocity"; initVeloc "Initial velocity"; samplePeriod "Sample period (sec)"
      mask help: Integrates acceleration twice to produce velocity and displacement. When clipping occurs, acceleration, velocity and displacement are adjusted accordingly.
  friction : Subsystem  Orientation=left  mask{friction=friction(id)*forceCanon, yieldDispl=yieldDispl(id)*lengthCanon, hysteresis=0}
      mask prompts: friction "Sliding friction"; yieldDispl "Equiv. yield displacement (in)"; hysteresis "Hysteresis constant"
  mass : Constant  Value=mass(id)*massCanon  OutDataType=sfix(16)  ConRadixGroup=Use specified scaling  OutScaling=2^0  SampleTime=inf  FramePeriod=inf
  spring : Gain  Orientation=left  Gain=spring(id)*springCanon
  static force : Constant  Value=staticForce(id)*forceCanon  OutDataType=sfix(16)  ConRadixGroup=Use specified scaling  OutScaling=2^0  SampleTime=inf  FramePeriod=inf
  term1 : Terminator
  unit dly : UnitDelay  Orientation=left  SampleTime=-1
  veloc units : Gain  Gain=1/velocCanon
  displ : Outport
  veloc : Outport  Port=2
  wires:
  double integrator/2 -> friction/1(veloc), veloc units/1
  double integrator/1 -> unit dly/1, displ/1
  div/1 -> double integrator/1
  double integrator/3 -> term1/1
  spring/1 -> Sum/3  "spring force"
  mass/1 -> div/2
  force/1 -> Sum/1  "total force"
  static force/1 -> Sum/4  "static force"
  Sum/1 -> div/1  "inertial force"
  veloc units/1 -> veloc/1
  unit dly/1 -> spring/1
  friction/1(force) -> Sum/2  "friction force"

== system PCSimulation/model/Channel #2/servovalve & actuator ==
  note: Parameter vector: 1: oil bulk modulus (force/displ^2) 2: servovalve delay (sec) 3: servovalve overlap 4: rated pressure (force/displ^2) 5: rated flow at rated pressure (displ^3/sec) 6: nominal flow at rated pressure (displ^3/sec) 7: actuator piston area 1 (displ^2) 8: actuator piston area 2 (displ^2) 9: actuator usable stroke 1 (displ) 10: actuator usable stroke 2 (displ) 11: actuator end cushion length 1 (displ) 12: actuator end cushion length 2 (displ) 13: additional port volume 1 (displ^3) 14: additional port volume 1 (displ^3) 15: actuator parasitic damping factor 16: cross-chamber leakage factor (flow/press) 17: ratio port openings according to area 18: sample period (sec) Conversion factors used for converting signals from external (user) to internal (canonical) units: 19: displacement 20: velocity 21: force 22: pressure 23: flow
  note: Note: "1" and "2" denote actuator cylinders on either side of the actuator piston. With positive valve drive, oil is ported into cylinder 1, resulting in positive displacement.
  note: Auxiliary diagnostic output vector: 1: valve opening 2: C1 pressure 3: C2 pressure 4: delta pressure 5: force 6: velocity 7: C1 flow 8: C2 flow 9: total flow 10: kinematic flow 11: compressibility flow 12: leakage flow 13: C1 oilspring displacement 14: C2 oilspring displacement 15: C1 oilspring velocity 16: C2 oilspring velocity
  cmd : Inport
  displ : Inport  Port=2
  veloc : Inport  Port=3
  spl press : Inport  Port=4
  rtn press : Inport  Port=5
  abs : Abs  SaturateOnIntegerOverflow=on  SampleTime=-1
  actuator : S-Function  FunctionName=Actuator  Parameters=params
  total flow sel : Selector  InputType=Vector  ElementSrc=Internal  Elements=9  RowSrc=Internal  Rows=1  ColumnSrc=Internal  Columns=1  IndexIsStartValue=off
  force : Outport
  flow : Outport  Port=2
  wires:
  spl press/1 -> actuator/4
  rtn press/1 -> actuator/5
  cmd/1 -> actuator/1
  actuator/1 -> force/1
  displ/1 -> actuator/2
  veloc/1 -> actuator/3
  actuator/2 -> total flow sel/1
  total flow sel/1 -> abs/1
  abs/1 -> flow/1

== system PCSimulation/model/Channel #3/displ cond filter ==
  inp : Inport
  filter : DiscreteFilter  Numerator=b  Denominator=a  SampleTime=-1
  out : Outport
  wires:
  inp/1 -> filter/1
  filter/1 -> out/1

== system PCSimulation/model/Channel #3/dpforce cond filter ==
  inp : Inport
  filter : DiscreteFilter  Numerator=b  Denominator=a  SampleTime=-1
  out : Outport
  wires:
  filter/1 -> out/1
  inp/1 -> filter/1

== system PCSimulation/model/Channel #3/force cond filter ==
  inp : Inport
  filter : DiscreteFilter  Numerator=b  Denominator=a  SampleTime=-1
  out : Outport
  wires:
  inp/1 -> filter/1
  filter/1 -> out/1

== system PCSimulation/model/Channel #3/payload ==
  force : Inport
  Sum : Sum  Inputs=+---
  div : Product  Inputs=*/
  double integrator : S-Function  FunctionName=doubleintegrator  Parameters=maxDispl, minDispl, initDispl, maxVeloc, minVeloc, initVeloc, samplePeriod  mask(Double integrator){maxDispl=maxDispl(id), minDispl=minDispl(id), initDispl=0, maxVeloc=maxVeloc(id)*velocCanon, minVeloc=minVeloc(id)*velocCanon, initVeloc=0, samplePeriod=samplePeriod}
      mask prompts: maxDispl "Maximum displacement"; minDispl "Minimum displacement"; initDispl "Initial displacement"; maxVeloc "Maximum velocity"; minVeloc "Minimum velocity"; initVeloc "Initial velocity"; samplePeriod "Sample period (sec)"
      mask help: Integrates acceleration twice to produce velocity and displacement. When clipping occurs, acceleration, velocity and displacement are adjusted accordingly.
  friction : Subsystem  Orientation=left  mask{friction=friction(id)*forceCanon, yieldDispl=yieldDispl(id)*lengthCanon, hysteresis=0}
      mask prompts: friction "Sliding friction"; yieldDispl "Equiv. yield displacement (in)"; hysteresis "Hysteresis constant"
  mass : Constant  Value=mass(id)*massCanon  OutDataType=sfix(16)  ConRadixGroup=Use specified scaling  OutScaling=2^0  SampleTime=inf  FramePeriod=inf
  spring : Gain  Orientation=left  Gain=spring(id)*springCanon
  static force : Constant  Value=staticForce(id)*forceCanon  OutDataType=sfix(16)  ConRadixGroup=Use specified scaling  OutScaling=2^0  SampleTime=inf  FramePeriod=inf
  term1 : Terminator
  unit dly : UnitDelay  Orientation=left  SampleTime=-1
  veloc units : Gain  Gain=1/velocCanon
  displ : Outport
  veloc : Outport  Port=2
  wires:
  friction/1(force) -> Sum/2  "friction force"
  unit dly/1 -> spring/1
  veloc units/1 -> veloc/1
  Sum/1 -> div/1  "inertial force"
  static force/1 -> Sum/4  "static force"
  force/1 -> Sum/1  "total force"
  mass/1 -> div/2
  spring/1 -> Sum/3  "spring force"
  double integrator/3 -> term1/1
  div/1 -> double integrator/1
  double integrator/1 -> displ/1, unit dly/1
  double integrator/2 -> veloc units/1, friction/1(veloc)

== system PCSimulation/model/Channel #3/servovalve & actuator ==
  note: Auxiliary diagnostic output vector: 1: valve opening 2: C1 pressure 3: C2 pressure 4: delta pressure 5: force 6: velocity 7: C1 flow 8: C2 flow 9: total flow 10: kinematic flow 11: compressibility flow 12: leakage flow 13: C1 oilspring displacement 14: C2 oilspring displacement 15: C1 oilspring velocity 16: C2 oilspring velocity
  note: Note: "1" and "2" denote actuator cylinders on either side of the actuator piston. With positive valve drive, oil is ported into cylinder 1, resulting in positive displacement.
  note: Parameter vector: 1: oil bulk modulus (force/displ^2) 2: servovalve delay (sec) 3: servovalve overlap 4: rated pressure (force/displ^2) 5: rated flow at rated pressure (displ^3/sec) 6: nominal flow at rated pressure (displ^3/sec) 7: actuator piston area 1 (displ^2) 8: actuator piston area 2 (displ^2) 9: actuator usable stroke 1 (displ) 10: actuator usable stroke 2 (displ) 11: actuator end cushion length 1 (displ) 12: actuator end cushion length 2 (displ) 13: additional port volume 1 (displ^3) 14: additional port volume 1 (displ^3) 15: actuator parasitic damping factor 16: cross-chamber leakage factor (flow/press) 17: ratio port openings according to area 18: sample period (sec) Conversion factors used for converting signals from external (user) to internal (canonical) units: 19: displacement 20: velocity 21: force 22: pressure 23: flow
  cmd : Inport
  displ : Inport  Port=2
  veloc : Inport  Port=3
  spl press : Inport  Port=4
  rtn press : Inport  Port=5
  abs : Abs  SaturateOnIntegerOverflow=on  SampleTime=-1
  actuator : S-Function  FunctionName=Actuator  Parameters=params
  total flow sel : Selector  InputType=Vector  ElementSrc=Internal  Elements=9  RowSrc=Internal  Rows=1  ColumnSrc=Internal  Columns=1  IndexIsStartValue=off
  force : Outport
  flow : Outport  Port=2
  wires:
  abs/1 -> flow/1
  total flow sel/1 -> abs/1
  actuator/2 -> total flow sel/1
  veloc/1 -> actuator/3
  displ/1 -> actuator/2
  actuator/1 -> force/1
  cmd/1 -> actuator/1
  rtn press/1 -> actuator/5
  spl press/1 -> actuator/4

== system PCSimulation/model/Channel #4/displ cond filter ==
  inp : Inport
  filter : DiscreteFilter  Numerator=b  Denominator=a  SampleTime=-1
  out : Outport
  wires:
  filter/1 -> out/1
  inp/1 -> filter/1

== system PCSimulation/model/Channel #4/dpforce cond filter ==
  inp : Inport
  filter : DiscreteFilter  Numerator=b  Denominator=a  SampleTime=-1
  out : Outport
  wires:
  inp/1 -> filter/1
  filter/1 -> out/1

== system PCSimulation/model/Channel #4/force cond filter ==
  inp : Inport
  filter : DiscreteFilter  Numerator=b  Denominator=a  SampleTime=-1
  out : Outport
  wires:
  filter/1 -> out/1
  inp/1 -> filter/1

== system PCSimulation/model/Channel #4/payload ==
  force : Inport
  Sum : Sum  Inputs=+---
  div : Product  Inputs=*/
  double integrator : S-Function  FunctionName=doubleintegrator  Parameters=maxDispl, minDispl, initDispl, maxVeloc, minVeloc, initVeloc, samplePeriod  mask(Double integrator){maxDispl=maxDispl(id), minDispl=minDispl(id), initDispl=0, maxVeloc=maxVeloc(id)*velocCanon, minVeloc=minVeloc(id)*velocCanon, initVeloc=0, samplePeriod=samplePeriod}
      mask prompts: maxDispl "Maximum displacement"; minDispl "Minimum displacement"; initDispl "Initial displacement"; maxVeloc "Maximum velocity"; minVeloc "Minimum velocity"; initVeloc "Initial velocity"; samplePeriod "Sample period (sec)"
      mask help: Integrates acceleration twice to produce velocity and displacement. When clipping occurs, acceleration, velocity and displacement are adjusted accordingly.
  friction : Subsystem  Orientation=left  mask{friction=friction(id)*forceCanon, yieldDispl=yieldDispl(id)*lengthCanon, hysteresis=0}
      mask prompts: friction "Sliding friction"; yieldDispl "Equiv. yield displacement (in)"; hysteresis "Hysteresis constant"
  mass : Constant  Value=mass(id)*massCanon  OutDataType=sfix(16)  ConRadixGroup=Use specified scaling  OutScaling=2^0  SampleTime=inf  FramePeriod=inf
  spring : Gain  Orientation=left  Gain=spring(id)*springCanon
  static force : Constant  Value=staticForce(id)*forceCanon  OutDataType=sfix(16)  ConRadixGroup=Use specified scaling  OutScaling=2^0  SampleTime=inf  FramePeriod=inf
  term1 : Terminator
  unit dly : UnitDelay  Orientation=left  SampleTime=-1
  veloc units : Gain  Gain=1/velocCanon
  displ : Outport
  veloc : Outport  Port=2
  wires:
  double integrator/2 -> friction/1(veloc), veloc units/1
  double integrator/1 -> unit dly/1, displ/1
  div/1 -> double integrator/1
  double integrator/3 -> term1/1
  spring/1 -> Sum/3  "spring force"
  mass/1 -> div/2
  force/1 -> Sum/1  "total force"
  static force/1 -> Sum/4  "static force"
  Sum/1 -> div/1  "inertial force"
  veloc units/1 -> veloc/1
  unit dly/1 -> spring/1
  friction/1(force) -> Sum/2  "friction force"

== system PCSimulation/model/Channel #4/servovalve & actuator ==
  note: Parameter vector: 1: oil bulk modulus (force/displ^2) 2: servovalve delay (sec) 3: servovalve overlap 4: rated pressure (force/displ^2) 5: rated flow at rated pressure (displ^3/sec) 6: nominal flow at rated pressure (displ^3/sec) 7: actuator piston area 1 (displ^2) 8: actuator piston area 2 (displ^2) 9: actuator usable stroke 1 (displ) 10: actuator usable stroke 2 (displ) 11: actuator end cushion length 1 (displ) 12: actuator end cushion length 2 (displ) 13: additional port volume 1 (displ^3) 14: additional port volume 1 (displ^3) 15: actuator parasitic damping factor 16: cross-chamber leakage factor (flow/press) 17: ratio port openings according to area 18: sample period (sec) Conversion factors used for converting signals from external (user) to internal (canonical) units: 19: displacement 20: velocity 21: force 22: pressure 23: flow
  note: Note: "1" and "2" denote actuator cylinders on either side of the actuator piston. With positive valve drive, oil is ported into cylinder 1, resulting in positive displacement.
  note: Auxiliary diagnostic output vector: 1: valve opening 2: C1 pressure 3: C2 pressure 4: delta pressure 5: force 6: velocity 7: C1 flow 8: C2 flow 9: total flow 10: kinematic flow 11: compressibility flow 12: leakage flow 13: C1 oilspring displacement 14: C2 oilspring displacement 15: C1 oilspring velocity 16: C2 oilspring velocity
  cmd : Inport
  displ : Inport  Port=2
  veloc : Inport  Port=3
  spl press : Inport  Port=4
  rtn press : Inport  Port=5
  abs : Abs  SaturateOnIntegerOverflow=on  SampleTime=-1
  actuator : S-Function  FunctionName=Actuator  Parameters=params
  total flow sel : Selector  InputType=Vector  ElementSrc=Internal  Elements=9  RowSrc=Internal  Rows=1  ColumnSrc=Internal  Columns=1  IndexIsStartValue=off
  force : Outport
  flow : Outport  Port=2
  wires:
  spl press/1 -> actuator/4
  rtn press/1 -> actuator/5
  cmd/1 -> actuator/1
  actuator/1 -> force/1
  displ/1 -> actuator/2
  veloc/1 -> actuator/3
  actuator/2 -> total flow sel/1
  total flow sel/1 -> abs/1
  abs/1 -> flow/1

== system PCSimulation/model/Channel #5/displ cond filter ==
  inp : Inport
  filter : DiscreteFilter  Numerator=b  Denominator=a  SampleTime=-1
  out : Outport
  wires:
  inp/1 -> filter/1
  filter/1 -> out/1

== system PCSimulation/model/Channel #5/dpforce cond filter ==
  inp : Inport
  filter : DiscreteFilter  Numerator=b  Denominator=a  SampleTime=-1
  out : Outport
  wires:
  filter/1 -> out/1
  inp/1 -> filter/1

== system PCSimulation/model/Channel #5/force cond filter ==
  inp : Inport
  filter : DiscreteFilter  Numerator=b  Denominator=a  SampleTime=-1
  out : Outport
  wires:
  inp/1 -> filter/1
  filter/1 -> out/1
